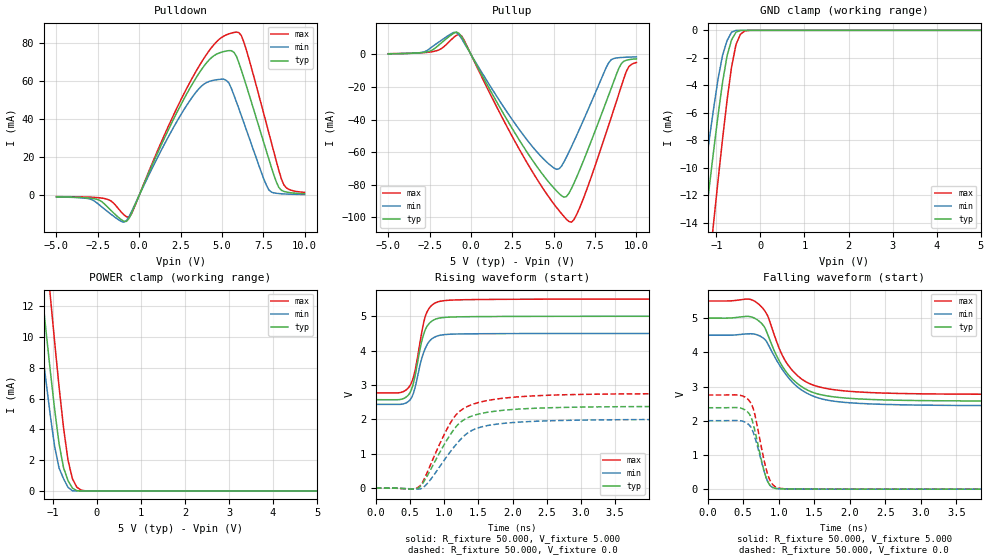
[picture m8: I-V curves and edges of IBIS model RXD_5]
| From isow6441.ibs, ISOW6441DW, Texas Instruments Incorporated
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|   RXD_5 Model
[Model]   RXD_5
Model_type 3-state
| Signals   RXD
Vmeas = 2.2V   |Reference voltage for timing measurements
Cref = 15pF   |Timing specification test load capacitance value
Vref = 0   |Timing specification test load voltage; GND
Polarity   Non-Inverting
Enable   Active-High
C_comp   2.100pF   1.700pF   2.500pF
[Temperature Range]   27.000   -40.000   0.125k
[Voltage Range]   5.000V   4.500V   5.500V
[Pullup Reference]   5.000V   4.500V   5.500V
[Pulldown Reference]   0.0V   0.0V   0.0V
[POWER Clamp Reference]   5.000V   4.500V   5.500V
[GND Clamp Reference]   0.0V   0.0V   0.0V
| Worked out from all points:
|   slope of the pulldown table from 0 to 0.75 V, typ, clamps not added: 49.4 ohm
|   slope of the pullup table from 0 to 0.75 V, typ, clamps not added: 52.4 ohm
|   GND clamp passes 1 mA (typ) near -0.68 V on its own axis
|   POWER clamp passes 1 mA (typ) near -0.70 V on its own axis
|   rising waveform, R_fixture 50.000, V_fixture 5.000: 20-80 % time 156ps typ, 166ps min, 155ps max; typ from 2.57 V to 5 V
|   rising waveform, R_fixture 50.000, V_fixture 0.0: 20-80 % time 446ps typ, 486ps min, 436ps max; typ from 0 V to 2.38 V
|   falling waveform, R_fixture 50.000, V_fixture 5.000: 20-80 % time 435ps typ, 472ps min, 401ps max; typ from 5 V to 2.57 V
|   falling waveform, R_fixture 50.000, V_fixture 0.0: 20-80 % time 160ps typ, 161ps min, 166ps max; typ from 2.38 V to 0 V
[Pulldown]
|Voltage   I(typ)   I(min)   I(max)
-5V       -789.1uA   -841.8uA   -673.3uA
-1.98V    -5.54mA    -8.044mA   -1.917mA
-621mV    -12.29mA   -11.38mA   -11.49mA
1.795V    35.02mA    31.31mA    36.96mA
3.607V    64.14mA    56.09mA    67.82mA
5.117V    75.68mA    61.15mA    83.84mA
5.872V    73.32mA    49.31mA    85.93mA
6.325V    61.88mA    38.26mA    80.73mA
7.684V    23.41mA    5.495mA    37.9mA
8.439V    4.187mA    938.4uA    13.18mA
8.892V    1.732mA    682.5uA    3.977mA
10V       852.9uA    423uA      1.516mA
[Pullup]
|Voltage   I(typ)   I(min)   I(max)
-5V       417uA      346.5uA    464.4uA
-2.231V   3.391mA    5.539mA    1.9mA
-1.023V   13.15mA    13.58mA    10.61mA
-570mV    10.88mA    9.81mA     11.4mA
4.413V    -74.71mA   -64.47mA   -83.19mA
5.319V    -85.31mA   -70.27mA   -95.84mA
6.074V    -82.33mA   -56.63mA   -103mA
6.829V    -64.52mA   -39.65mA   -87.54mA
8.339V    -24.54mA   -4.894mA   -42.94mA
9.094V    -5.547mA   -1.864mA   -19.31mA
9.547V    -3.211mA   -1.63mA    -7.435mA
10V       -2.699mA   -1.501mA   -4.94mA
[GND_clamp]
|Voltage   I(typ)   I(min)   I(max)
-5V       -121.9mA   -103.6mA   -144.6mA
-1.465V   -19.77mA   -15.18mA   -26.74mA
-1.364V   -16.95mA   -12.73mA   -23.49mA
-1.263V   -14.15mA   -10.31mA   -20.26mA
-1.061V   -8.696mA   -5.622mA   -13.91mA
-859mV    -3.742mA   -1.796mA   -7.855mA
-758mV    -1.853mA   -749.3uA   -5.081mA
-657mV    -699uA     -138.4uA   -2.686mA
-556mV    -139.4uA   -3.674uA   -1.038mA
-455mV    -8.262uA   -24.17nA   -281.6uA
-354mV    -204.1nA   -188.5pA   -43.63uA
5V        0A         0A         0A
[POWER_clamp]
|Voltage   I(typ)   I(min)   I(max)
-5V       122.5mA    104mA      145.7mA
-1.464V   19.02mA    14.57mA    25.71mA
-1.363V   16.16mA    12.1mA     22.42mA
-1.262V   13.34mA    9.662mA    19.15mA
-1.06V    7.868mA    4.966mA    12.76mA
-959mV    5.305mA    2.886mA    9.684mA
-858mV    3.056mA    1.487mA    6.759mA
-757mV    1.51mA     796.4uA    4.108mA
-656mV    673.1uA    233.8uA    2.011mA
-555mV    180.8uA    12.8uA     787.7uA
-252mV    14.4nA     21.67pA    4.687uA
5V        0A         0A         0A
[Ramp]
| variable   typ   min   max
dV/dt_r   1.428/0.446n   1.202/0.486n   1.651/0.436n
dV/dt_f   1.456/0.434n   1.237/0.472n   1.638/0.400n
R_load = 50.000
[Rising Waveform]
R_fixture= 50.000
V_fixture= 5.000
V_fixture_min= 4.500
V_fixture_max= 5.500
|time   V(typ)   V(min)   V(max)
0s        2.573V     2.438V     2.771V
355ps     2.579V     2.438V     2.78V
480ps     2.72V      2.527V     2.928V
524ps     2.881V     2.64V      3.079V
561ps     3.145V     2.832V     3.308V
663ps     4.195V     3.713V     4.427V
739ps     4.671V     4.129V     5.078V
842ps     4.888V     4.373V     5.356V
1.022ns   4.969V     4.47V      5.459V
15ns      5V         4.5V       5.5V
[Rising Waveform]
R_fixture= 50.000
V_fixture= 0.0
V_fixture_min= 0.0
V_fixture_max= 0.0
|time   V(typ)   V(min)   V(max)
0s        641.2nV    230.8nV    1.647uV
615ps     2.336mV    -26.58mV   21.83mV
679ps     123.6mV    2.278mV    152.6mV
759ps     382.5mV    149.5mV    491.7mV
1.037ns   1.391V     916mV      1.703V
1.197ns   1.84V      1.324V     2.182V
1.477ns   2.142V     1.74V      2.478V
1.997ns   2.288V     1.908V     2.643V
4.047ns   2.375V     1.997V     2.746V
15ns      2.38V      2.003V     2.752V
[Falling Waveform]
R_fixture= 50.000
V_fixture= 5.000
V_fixture_min= 4.500
V_fixture_max= 5.500
|time   V(typ)   V(min)   V(max)
0s        5V         4.5V       5.5V
572ps     5.05V      4.541V     5.556V
673ps     4.983V     4.525V     5.479V
820ps     4.65V      4.342V     5.162V
1.05ns    3.598V     3.502V     3.917V
1.26ns    3.093V     2.994V     3.326V
1.54ns    2.788V     2.677V     3.005V
1.99ns    2.655V     2.526V     2.86V
3.89ns    2.577V     2.444V     2.775V
15ns      2.573V     2.438V     2.771V
[Falling Waveform]
R_fixture= 50.000
V_fixture= 0.0
V_fixture_min= 0.0
V_fixture_max= 0.0
|time   V(typ)   V(min)   V(max)
0s        2.38V      2.003V     2.752V
442ps     2.379V     2.005V     2.749V
580ps     2.216V     1.885V     2.597V
623ps     2.038V     1.76V      2.452V
661ps     1.745V     1.54V      2.213V
776ps     678.8mV    664.2mV    1.021V
842ps     238.5mV    239.7mV    450.8mV
927ps     38.91mV    38.79mV    111.7mV
1.057ns   8.766mV    6.963mV    16.24mV
15ns      927.5pV    592.6pV    107.7nV
